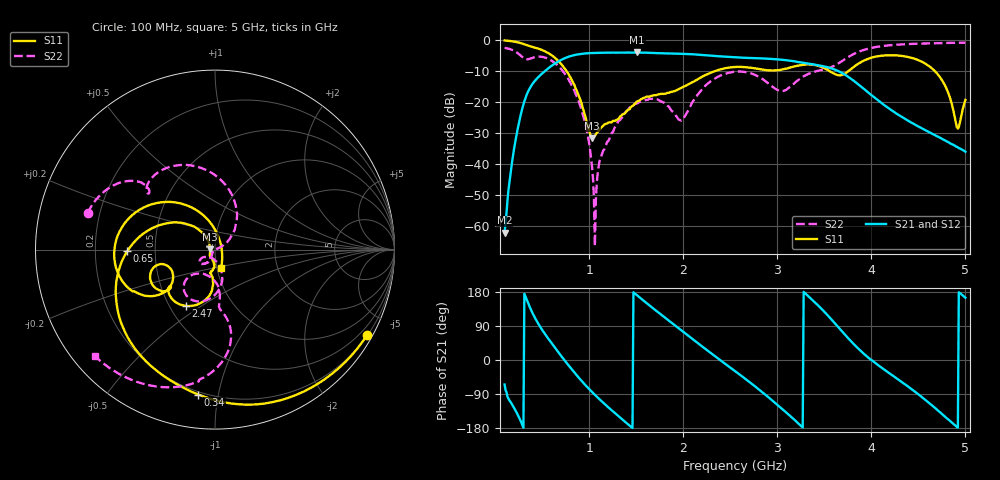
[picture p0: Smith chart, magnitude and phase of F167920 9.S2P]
!  2-Port S-parameters saved by WinCal
! VAR MeasName=S-Parameters (CALIBRATED_DATA) read from VNA (N5242A)
! VAR MeasDate=2016-11-22 9:53:59
! VAR NAME=F167920 9
! VAR FILENAME=F167920 9.S2P
! VAR DATE=2016-11-22 9:53:59
! VAR PHYS_PORTS=1,2
# Hz S DB R 50
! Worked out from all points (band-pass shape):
!   491 points, 100 MHz to 5 GHz, reference 50 ohm
!   highest |S21| = -4.12 dB at 1.51 GHz (marker M1); lowest = -62.0 dB at 100 MHz (marker M2)
!   |S21| within 3 dB of the highest: 664 MHz to 3.21 GHz (2.546 GHz wide, 131 % of centre)
!   lowest |S11| = -31.6 dB at 1.03 GHz (marker M3), VSWR 1.05, Z = 47.4 + j0.225 ohm
!   |S11| at or under -10 dB: 756.1 MHz to 2.345 GHz (1.589 GHz wide, 102 % of centre); 3.55 GHz to 3.76 GHz (209.7 MHz wide, 5.74 % of centre); 4.672 GHz to end of sweep
!   |S22| runs from -66.3 to -1.0 dB; largest |S21 - S12| = 0.0015
!   S11 on the Smith chart (normalised r, x): 100 MHz: 0.22, -3.82; 340 MHz: 0.18, -0.87; 650 MHz: 0.34, -0.01; 2.47 GHz: 0.60, -0.43; 5 GHz: 1.05, -0.22
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1e8  -0.25 -29.3  -62.03 -64.6  -61.32 -63.4  -2.64 163.9
2.1e8  -0.66 -60.8  -33.39 -130.9  -33.44 -130.5  -3.72 145.3
3.4e8  -1.80 -96.6  -17.30 156.1  -17.29 156.1  -6.32 139.6
6.5e8  -6.21 -179.0  -7.37 27.4  -7.36 27.4  -7.89 87.8
9.2e8  -20.59 124.0  -4.52 -55.5  -4.51 -55.5  -22.93 29.8
1.03e9  -31.60 174.8  -4.28 -84.6  -4.28 -84.5  -40.90 24.6
1.05e9  -31.23 -168.0  -4.27 -89.4  -4.27 -89.5  -50.98 19.8
1.07e9  -30.38 -155.9  -4.25 -94.3  -4.25 -94.3  -51.78 -141.1
1.1e9  -29.21 -144.1  -4.22 -101.4  -4.22 -101.4  -40.74 -147.7
1.15e9  -27.60 -132.5  -4.18 -113.1  -4.18 -113.1  -35.54 -142.4
1.51e9  -19.79 -93.8  -4.12 170.4  -4.12 170.4  -20.50 -125.9
1.74e9  -17.53 -100.9  -4.32 124.6  -4.31 124.6  -19.44 -144.0
1.98e9  -15.47 -93.7  -4.56 78.4  -4.56 78.4  -26.01 -110.6
2.47e9  -9.04 -117.4  -5.53 -14.5  -5.53 -14.5  -10.73 -101.3
2.55e9  -8.77 -124.4  -5.68 -29.2  -5.67 -29.2  -10.29 -110.0
2.93e9  -9.90 -140.6  -6.16 -103.4  -6.15 -103.4  -14.67 -131.4
3.37e9  -8.02 -155.1  -7.87 159.2  -7.86 159.1  -10.52 -85.3
3.77e9  -9.76 -140.5  -12.25 53.1  -12.24 53.0  -5.29 -81.3
4.19e9  -5.00 -173.0  -22.17 -34.7  -22.15 -34.8  -1.81 -109.0
4.68e9  -10.25 124.8  -30.68 -127.2  -30.77 -127.4  -1.12 -129.4
4.92e9  -28.56 8.2  -34.57 -178.5  -34.63 -178.9  -1.00 -136.4
5e9  -19.34 -71.6  -36.00 164.5  -35.96 165.4  -0.97 -138.5
